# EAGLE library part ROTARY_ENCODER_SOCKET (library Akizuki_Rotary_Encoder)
Akizuki RotaryEncoder RGB
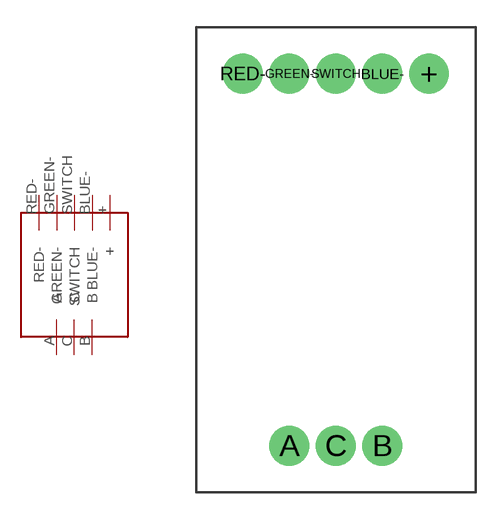
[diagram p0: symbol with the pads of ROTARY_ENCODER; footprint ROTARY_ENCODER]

Designator prefix CONNECTOR

## ROTARY_ENCODER_SOCKET  [ROTARY_ENCODER]
+  +
A  A
B  B
BLUE-  BLUE-
C  C
GREEN-  GREEN-
RED-  RED-
SWITCH  SWITCH

## Footprint ROTARY_ENCODER (pad centres in mm)
Akizuki Rotary Encoder RGB Rotary Encoder
drill 1 pad 2.184: + 5.08,20.32; A -2.54,0; B 2.54,0; BLUE- 2.54,20.32; C 0,0; GREEN- -2.54,20.32; RED- -5.08,20.32; SWITCH 0,20.32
